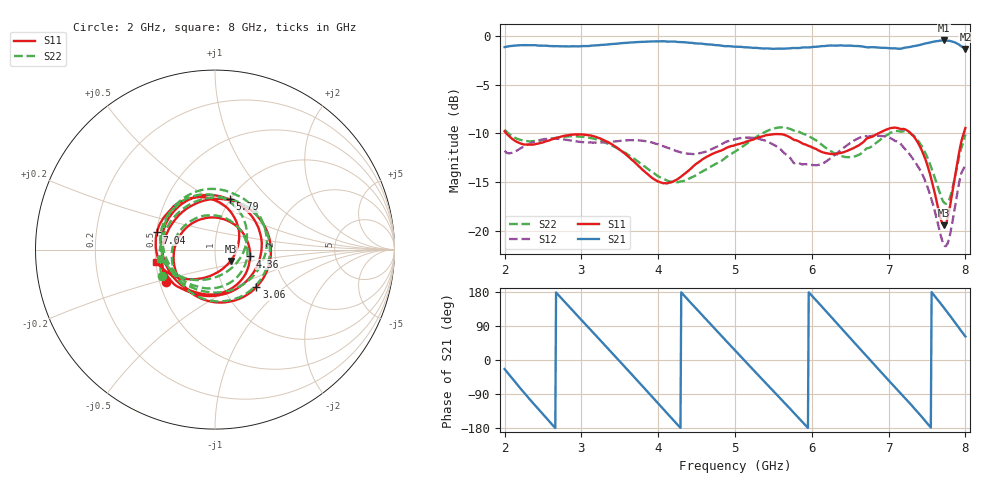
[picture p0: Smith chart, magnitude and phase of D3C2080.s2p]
! 11/4/2020 10:46:11 AM
! C:\USERS\DITOM\DESKTOP\SINGLE JUNCTION ISOLATOR DATA\2.0-8.0 GHZ (D3I2080).S2P
! CHANNEL.1
! TR.MEASUREMENT
! CORRECTED.DATA
# GHZ S RI R 50.0
! FREQ.GHZ  S11RE  S11IM  S21RE  S21IM  S12RE  S12IM  S22RE  S22IM
!; PortSelection: Port_12
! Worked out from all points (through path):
!   601 points, 2 GHz to 8 GHz, reference 50 ohm
!   highest |S21| = -0.49 dB at 7.72 GHz (marker M1); lowest = -1.4 dB at 8 GHz (marker M2)
!   lowest |S11| = -19.4 dB at 7.72 GHz (marker M3), VSWR 1.24, Z = 58.9 - j7.58 ohm
!   |S11| at or under -10 dB: 2.024 GHz to 6.864 GHz (4.84 GHz wide, 109 % of centre); 7.291 GHz to 7.977 GHz (686.6 MHz wide, 8.99 % of centre)
!   |S22| runs from -17.2 to -9.4 dB; largest |S21 - S12| = 0.86
!   S11 on the Smith chart (normalised r, x): 2 GHz: 0.54, -0.22; 3.06 GHz: 1.42, -0.66; 4.36 GHz: 1.48, -0.12; 5.79 GHz: 0.99, +0.61; 7.04 GHz: 0.50, +0.11; 8 GHz: 0.50, -0.08
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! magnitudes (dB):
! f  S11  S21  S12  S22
! 2 GHz  -9.8  -1.2  -11.8  -9.6
! 2.32 GHz  -11.1  -1.0  -11.1  -10.8
! 3 GHz  -10.1  -1.1  -10.9  -10.3
! 3.06 GHz  -10.2  -1.1  -10.9  -10.4
! 3.43 GHz  -11.3  -0.8  -10.8  -11.4
! 4 GHz  -14.9  -0.6  -11.1  -14.4
! 4.36 GHz  -14.0  -0.7  -12.0  -14.8
! 5 GHz  -11.2  -1.1  -10.6  -11.9
! 5.41 GHz  -10.2  -1.3  -10.8  -9.8
! 5.79 GHz  -10.7  -1.3  -13.0  -9.7
! 6 GHz  -11.4  -1.2  -13.2  -10.4
! 6.5 GHz  -11.6  -1.0  -11.0  -12.4
! 7 GHz  -9.5  -1.3  -10.4  -10.1
! 7.04 GHz  -9.4  -1.3  -10.6  -9.9
! 7.24 GHz  -9.7  -1.2  -11.8  -9.8
! 7.39 GHz  -11.1  -1.0  -13.4  -10.8
! 7.53 GHz  -13.9  -0.7  -16.0  -12.9
! 7.67 GHz  -18.5  -0.5  -20.2  -16.2
! 7.72 GHz  -19.4  -0.5  -21.4  -17.0
! 7.8 GHz  -17.4  -0.5  -20.3  -16.5
! 7.93 GHz  -11.5  -1.0  -14.6  -12.0
! 8 GHz  -9.4  -1.4  -13.2  -10.1
